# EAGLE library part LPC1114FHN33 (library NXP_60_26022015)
32-bit ARM Cortex-M0 microcontroller; up to 64 kB flash and 8 kB SRAM The LPC1110/11/12/13/14/15 are a ARM Cortex-M0 based, low-cost 32-bit MCU family, designed for 8/16-bit microcontroller applications, offering performance, low power, simple instruction set and memory addressing together with reduced code size compared to existing 8/16-bit architectures. The LPC1110/11/12/13/14/15 operate at CPU frequencies of up to 50 MHz. The peripheral complement of the LPC1110/11/12/13/14/15 includes up to 64 kB of flash memory, up to 8 kB of data memory, one Fast-mode Plus I 2 C-bus interface, one RS-485/EIA-485 UART, up to two SPI interfaces with SSP features, four general purpose counter/timers, a 10-bit ADC, and up to 42 general purpose I/O pins. Remark: The LPC111x series consists of the LPC1100 series (parts LPC111x/101/201/301), LPC1100L series (parts LPC111x/002/102/202/302), and the LPC1100XL series (parts LPC111x/103/203/303/323/333). The LPC1100L and LPC1100XL series include the power profiles, a windowed watchdog timer, and a configurable open-drain mode. AAL Eindhoven MK
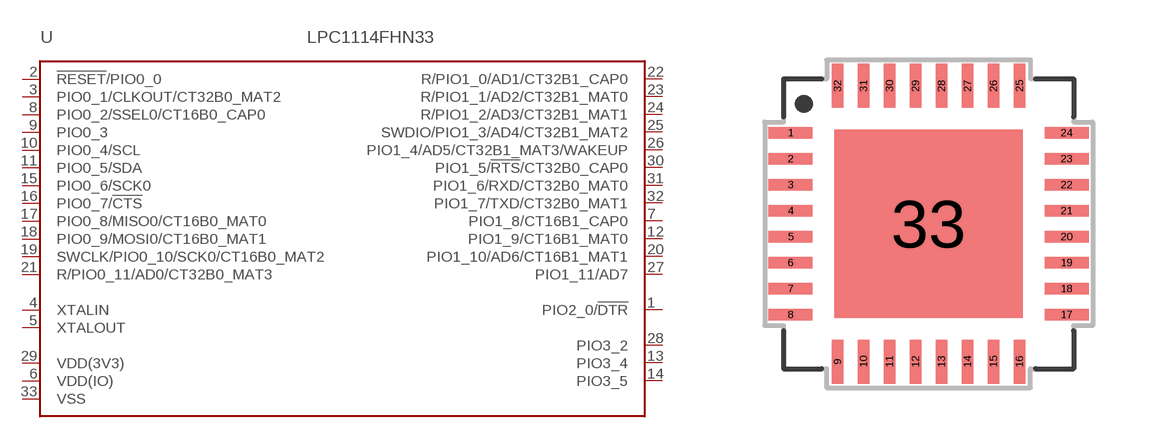
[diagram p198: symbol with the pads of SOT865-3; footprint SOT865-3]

Designator prefix U

## LPC1114FHN33/101 (ADC: 8; FLASH: 16kB; GPIO: 28; PWR_PROFILES: no; SERIES: LPC1100; SPI: 1; SRAM: 2kB), LPC1114FHN33/102 (ADC: 8; FLASH: 16kB; GPIO: 28; PWR_PROFILES: yes; SERIES: LPC1100L; SPI: 1; SRAM: 2kB), LPC1114FHN33/201 (ADC: 8; FLASH: 16kB; GPIO: 28; PWR_PROFILES: no; SERIES: LPC1100; SPI: 1; SRAM: 4kB), LPC1114FHN33/202 (ADC: 8; FLASH: 16KB; GPIO: 28; PWR_PROFILES: yes; SERIES: LPC1100L; SPI: 1; SRAM: 4kB)  [SOT865-3]
1  PIO2_0/!DTR!
2  !RESET!/PIO0_0
3  PIO0_1/CLKOUT/CT32B0_MAT2
4  XTALIN  in
5  XTALOUT  out
6  VDD(IO)  pwr
7  PIO1_8/CT16B1_CAP0
8  PIO0_2/SSEL0/CT16B0_CAP0
9  PIO0_3
10  PIO0_4/SCL
11  PIO0_5/SDA
12  PIO1_9/CT16B1_MAT0
13  PIO3_4
14  PIO3_5
15  PIO0_6/SCK0
16  PIO0_7/!CTS!
17  PIO0_8/MISO0/CT16B0_MAT0
18  PIO0_9/MOSI0/CT16B0_MAT1
19  SWCLK/PIO0_10/SCK0/CT16B0_MAT2
20  PIO1_10/AD6/CT16B1_MAT1
21  R/PIO0_11/AD0/CT32B0_MAT3
22  R/PIO1_0/AD1/CT32B1_CAP0
23  R/PIO1_1/AD2/CT32B1_MAT0
24  R/PIO1_2/AD3/CT32B1_MAT1
25  SWDIO/PIO1_3/AD4/CT32B1_MAT2
26  PIO1_4/AD5/CT32B1_MAT3/WAKEUP
27  PIO1_11/AD7
28  PIO3_2
29  VDD(3V3)  pwr
30  PIO1_5/!RTS!/CT32B0_CAP0
31  PIO1_6/RXD/CT32B0_MAT0
32  PIO1_7/TXD/CT32B0_MAT1
33  VSS  pwr

## Footprint SOT865-3 (pad centres in mm)
SOT865-3 HVQFN32: plastic thermal enhanced very thin quad flat package; no leads; 32 terminals; body 7 x 7 x 0.85 mm JEDEC: MO-220 IEC: -- JEITA: --
smd 1.1 x 0.28: 1 -3.45,2.275; 2 -3.45,1.625; 3 -3.45,0.975; 4 -3.45,0.325; 5 -3.45,-0.325; 6 -3.45,-0.975; 7 -3.45,-1.625; 8 -3.45,-2.275; 17 3.45,-2.275; 18 3.45,-1.625; 19 3.45,-0.975; 20 3.45,-0.325; 21 3.45,0.325; 22 3.45,0.975; 23 3.45,1.625; 24 3.45,2.275
smd 0.28 x 1.1: 9 -2.275,-3.45; 10 -1.625,-3.45; 11 -0.975,-3.45; 12 -0.325,-3.45; 13 0.325,-3.45; 14 0.975,-3.45; 15 1.625,-3.45; 16 2.275,-3.45; 25 2.275,3.45; 26 1.625,3.45; 27 0.975,3.45; 28 0.325,3.45; 29 -0.325,3.45; 30 -0.975,3.45; 31 -1.625,3.45; 32 -2.275,3.45
smd 4.7 x 4.7: 33 0,0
